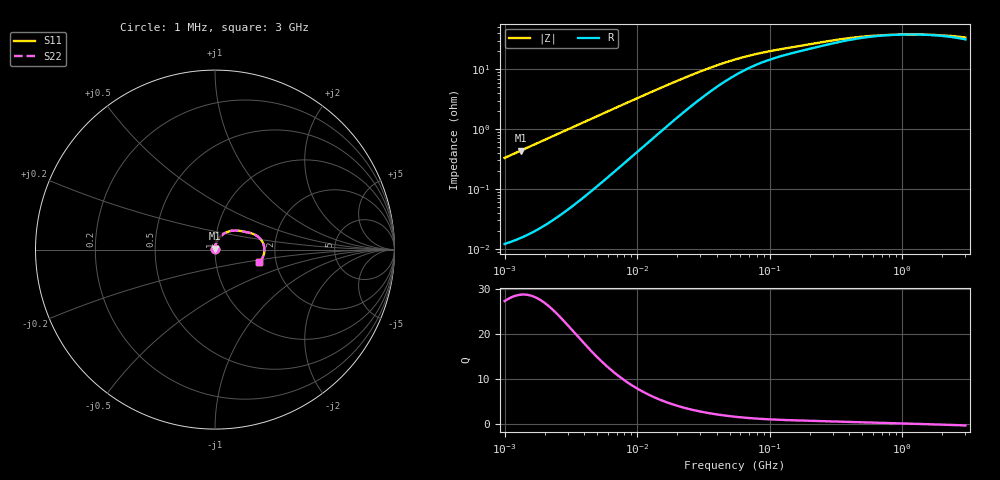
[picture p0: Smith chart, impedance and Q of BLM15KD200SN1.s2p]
! BLM15KD200SN1
# Hz S RI R 50
!Freq.(Hz) S11(Real) S11(Imag) S21(Real) S21(Imag) S12(Real) S12(Imag) S22(Real) S22(Imag)
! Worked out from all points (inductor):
!   401 points, 1 MHz to 3 GHz, reference 50 ohm
!   read as one part in series: L = 52.7 nH near 1.041 MHz
!   highest Q = 28.6 at 1.323 MHz (marker M1), where L = 52.7 nH
!   self-resonance near 1.146 GHz
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1000000  0.000133 0.00331  0.9999 -0.00331  0.9999 -0.00331  0.000133 0.00331
1040844  0.000137 0.00344  0.9999 -0.00344  0.9999 -0.00344  0.000137 0.00344
1323425  0.000172 0.00438  0.9998 -0.00438  0.9998 -0.00438  0.000172 0.00438
3823119  0.000845 0.0126  0.9992 -0.0126  0.9992 -0.0126  0.000845 0.0126
7858845  0.00327 0.0256  0.9967 -0.0256  0.9967 -0.0256  0.00327 0.0256
1.461624e7  0.0107 0.0458  0.9893 -0.0458  0.9893 -0.0458  0.0107 0.0458
2.181181e7  0.0221 0.0641  0.9779 -0.0641  0.9779 -0.0641  0.0221 0.0641
3.065274e7  0.039 0.0813  0.961 -0.0813  0.961 -0.0813  0.039 0.0813
4.138676e7  0.0604 0.0949  0.9396 -0.0949  0.9396 -0.0949  0.0604 0.0949
5.477226e7  0.0849 0.1034  0.9151 -0.1034  0.9151 -0.1034  0.0849 0.1034
7.105049e7  0.109 0.1063  0.891 -0.1063  0.891 -0.1063  0.109 0.1063
9.216659e7  0.132 0.1051  0.868 -0.1051  0.868 -0.1051  0.132 0.1051
1.219755e8  0.1542 0.1015  0.8458 -0.1015  0.8458 -0.1015  0.1542 0.1015
2.094008e8  0.194 0.0932  0.806 -0.0932  0.806 -0.0932  0.194 0.0932
3.062963e8  0.2232 0.0826  0.7768 -0.0826  0.7768 -0.0826  0.2232 0.0826
4.135554e8  0.2441 0.0683  0.7559 -0.0683  0.7559 -0.0683  0.2441 0.0683
5.696638e8  0.261 0.0485  0.739 -0.0485  0.739 -0.0485  0.261 0.0485
8.005644e8  0.2716 0.0253  0.7284 -0.0253  0.7284 -0.0253  0.2716 0.0253
1.147801e9  0.2754 -0.000103  0.7246 0.000103  0.7246 0.000103  0.2754 -0.000103
1.645649e9  0.2721 -0.0261  0.7279 0.0261  0.7279 0.0261  0.2721 -0.0261
2.221924e9  0.263 -0.0485  0.737 0.0485  0.737 0.0485  0.263 -0.0485
3e9  0.246 -0.0707  0.754 0.0707  0.754 0.0707  0.246 -0.0707
